{attribute 'no_assign'}
FUNCTION_BLOCK FB_DO_IED_MUnn_LLN0_Mod EXTENDS FB_AcsiCommonControllableDataClass
VAR_INPUT
	stVal: FB_AcsiDATypeMod := (Fc:=ACSI_FC_ST, TrgOp:=ACSI_TrgOp_dchg, bLinkResult:=THIS^.AddDataToContainer(ipData:=stVal));
	q: FB_AcsiDATypeQuality := (Fc:=ACSI_FC_ST, TrgOp:=ACSI_TrgOp_qchg, bLinkResult:=THIS^.AddDataToContainer(ipData:=q));
	t: FB_AcsiDATypeTimeStamp := (Fc:=ACSI_FC_ST, bLinkResult:=THIS^.AddDataToContainer(ipData:=t));
	ctlModel: FB_AcsiDATypeCtlModels := (Fc:=ACSI_FC_CF, TrgOp:=ACSI_TrgOp_dchg, eValue:=E_AcsiCtlModels.StatusOnly, bLinkResult:=THIS^.AddDataToContainer(ipData:=ctlModel));
	
	fbControl: FB_DirectControl := (ipCtrl:=THIS^.AddServerJob(ipEvent:=fbControl, ipCompletion:=fbControl));
END_VAR
VAR
END_VAR

END_FUNCTION_BLOCK
